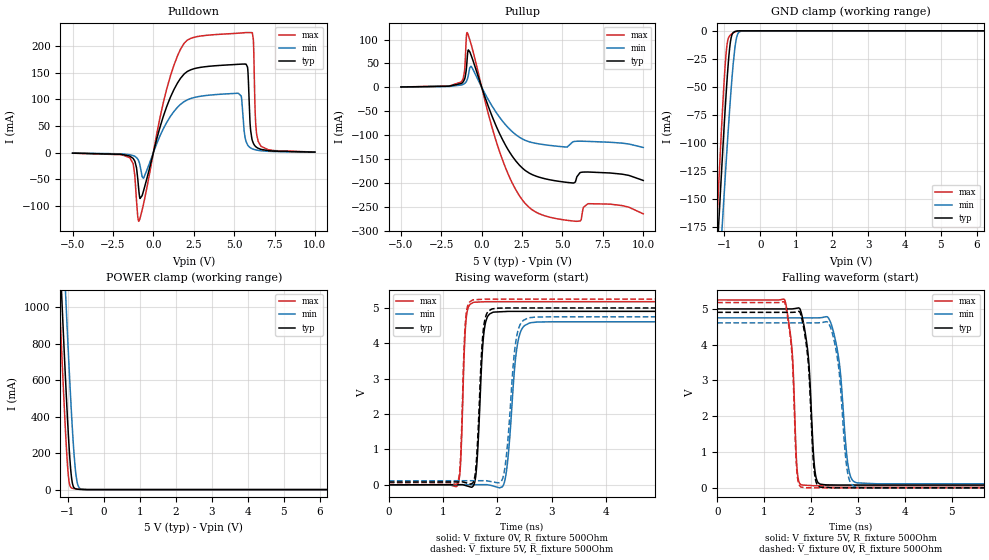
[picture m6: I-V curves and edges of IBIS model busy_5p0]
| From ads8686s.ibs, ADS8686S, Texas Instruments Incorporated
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|   busy_5p0 Model
[Model]   busy_5p0
Model_type   3-state
Polarity   Non-Inverting
Vmeas = 2.5
Vref = 2.5
Cref = 15pF
Rref = 50
|   typ   min   max
C_comp   1.49pF   1.49pF   1.52pF
[Voltage Range]   5   4.75   5.25
[Temperature Range]   27   125   -40
[Pullup Reference]   5   4.75   5.25
[Pulldown Reference]   0   0   0
[Power Clamp Reference]   5   4.75   5.25
[GND Clamp Reference]   0   0   0
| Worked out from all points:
|   slope of the pulldown table from 0 to 0.75 V, typ, clamps not added: 9.41 ohm
|   slope of the pullup table from 0 to 0.75 V, typ, clamps not added: 10.8 ohm
|   GND clamp passes 1 mA (typ) near -0.73 V on its own axis
|   POWER clamp passes 1 mA (typ) near -0.63 V on its own axis
|   falling waveform, V_fixture 5V, R_fixture 500Ohm: 20-80 % time 134ps typ, 188ps min, 110ps max; typ from 5 V to 0.078 V
|   rising waveform, V_fixture 0V, R_fixture 500Ohm: 20-80 % time 92ps typ, 139ps min, 66.5ps max; typ from 0 V to 4.9 V
|   rising waveform, V_fixture 5V, R_fixture 500Ohm: 20-80 % time 90.9ps typ, 140ps min, 65.1ps max; typ from 0.078 V to 5 V
|   falling waveform, V_fixture 0V, R_fixture 500Ohm: 20-80 % time 131ps typ, 178ps min, 108ps max; typ from 4.9 V to 0 V
[Pulldown]
|   Voltage   I(typ)   I(min)   I(max)
-5V       -801.1uA   -630.2uA   -897.9uA
-1.46V    -6.363mA   -3.781mA   -9.289mA
-905mV    -68.79mA   -15.37mA   -128.5mA
-605mV    -71.26mA   -47.34mA   -95.77mA
1.69V     139.6mA    90.76mA    194.3mA
5.26V     165.6mA    111.4mA    223.9mA
5.83V     160.4mA    14.88mA    225.1mA
5.995V    51.94mA    9.475mA    225.1mA
6.19V     17.76mA    6.551mA    212.4mA
6.31V     12.26mA    5.49mA     70.73mA
6.49V     8.288mA    4.409mA    21.24mA
10V       1.09mA     890.4uA    1.248mA
[GND Clamp]
|   Voltage   I(typ)   I(min)   I(max)
-5V       -2.651A    -2.459A    -2.919A
-1.25V    -227.9mA   -277.2mA   -199.5mA
-1.16V    -173.5mA   -227.8mA   -138.9mA
-1.07V    -120.6mA   -179.2mA   -81.19mA
-1.04V    -103.6mA   -163.3mA   -63.21mA
-980mV    -70.77mA   -132mA     -31.32mA
-935mV    -48.03mA   -109.2mA   -14.4mA
-830mV    -9.335mA   -59.33mA   -3.628mA
-710mV    -611.3uA   -15.52mA   -1.065mA
-635mV    -148.8uA   -3.228mA   -313.9uA
-515mV    -11.53uA   -121.6uA   -20.17uA
10V       0A         0A         0A
[Pullup]
|   Voltage   I(typ)   I(min)   I(max)
-5V       649.4uA    529.6uA    697.9uA
-1.25V    8.027mA    4.811mA    11.26mA
-1.07V    16.36mA    7.7mA      32.42mA
-950mV    38.79mA    12.34mA    106.1mA
-905mV    57.63mA    15.57mA    114.6mA
-830mV    78.38mA    24.81mA    109mA
-650mV    66.47mA    43.66mA    89.28mA
1.09V     -95.8mA    -62.03mA   -133.1mA
2.74V     -175.2mA   -111.7mA   -244.9mA
5.8V      -198.1mA   -113.1mA   -280.4mA
6.58V     -177.3mA   -113.3mA   -243.6mA
10V       -195mA     -126mA     -265mA
[POWER Clamp]
|   Voltage   I(typ)   I(min)   I(max)
-5V       19.86A     20.28A     19.6A
-1.25V    1.445A     1.936A     1.139A
-1.175V   1.105A     1.595A     800.1mA
-1.13V    905.9mA    1.393A     603.8mA
-1.07V    649.3mA    1.129A     357.7mA
-1.04V    526.6mA    999.9mA    246.4mA
-965mV    249.6mA    689mA      49.59mA
-875mV    42.07mA    353.9mA    7.605mA
-770mV    3.718mA    82.23mA    4.001mA
-710mV    1.997mA    21.42mA    2.636mA
-620mV    842.4uA    2.379mA    1.097mA
10V       0A         0A         0A
[Ramp]
R_load = 500
|   typ   min   max
dV/dt_r   2.94249/9.19736e-11   2.76609/1.3851e-10   3.10663/6.64669e-11
dV/dt_f   2.95306/1.34312e-10   2.78252/1.87919e-10   3.11407/1.10282e-10
[Falling Waveform]
V_fixture = 5V
V_fixture_min = 4.75V
V_fixture_max = 5.25V
R_fixture = 500Ohm
C_fixture = 0F
|   Time   V(typ)   V(min)   V(max)
0s        5V         4.75V      5.25V
1.436ns   4.999V     4.749V     5.259V
1.595ns   4.999V     4.749V     3.846V
1.692ns   5.019V     4.749V     726.9mV
1.791ns   4.894V     4.749V     85.5mV
2.186ns   109mV      4.753V     60.1mV
2.525ns   79.7mV     4.093V     60.09mV
2.778ns   78.38mV    721.2mV    60.08mV
2.957ns   78.37mV    147.2mV    60.08mV
10ns      78.24mV    112.5mV    59.88mV
[Rising Waveform]
V_fixture = 0V
V_fixture_min = 0V
V_fixture_max = 0V
R_fixture = 500Ohm
C_fixture = 0F
|   Time   V(typ)   V(min)   V(max)
0s        -92.52nV   -75.11nV   -36.98nV
1.27ns    3.674mV    2.938mV    2.092mV
1.419ns   -22.42mV   3.282mV    4.599V
1.555ns   -31.25mV   3.598mV    5.157V
1.747ns   4.248V     4.042mV    5.174V
1.912ns   4.876V     -29.77mV   5.178V
2.14ns    4.899V     148.1mV    5.178V
2.354ns   4.904V     3.83V      5.178V
2.588ns   4.904V     4.573V     5.178V
10ns      4.904V     4.61V      5.178V
[Rising Waveform]
V_fixture = 5V
V_fixture_min = 4.75V
V_fixture_max = 5.25V
R_fixture = 500Ohm
C_fixture = 0F
|   Time   V(typ)   V(min)   V(max)
0s        78.24mV    112.5mV    59.88mV
1.263ns   81.78mV    115.3mV    47.97mV
1.411ns   61.68mV    115.6mV    4.616V
1.544ns   49.81mV    115.9mV    5.226V
1.739ns   4.362V     116.4mV    5.247V
1.893ns   4.967V     88.36mV    5.25V
2.118ns   4.998V     306mV      5.25V
2.337ns   5V         4.039V     5.25V
2.555ns   5V         4.711V     5.25V
10ns      5V         4.75V      5.25V
[Falling Waveform]
|Gnd
V_fixture = 0V
V_fixture_min = 0V
V_fixture_max = 0V
R_fixture = 500Ohm
C_fixture = 0F
|   Time   V(typ)   V(min)   V(max)
0s        4.904V     4.61V      5.178V
1.436ns   4.903V     4.609V     5.186V
1.581ns   4.903V     4.609V     3.939V
1.692ns   4.916V     4.609V     555.3mV
1.778ns   4.851V     4.609V     28.91mV
2.167ns   35.19mV    4.612V     185.8uV
2.498ns   1.636mV    4.077V     177.9uV
2.76ns    295.3uV    588.5mV    171.7uV
2.929ns   288.4uV    32.71mV    167.7uV
10ns      -77.4nV    13.78nV    -36.34nV
